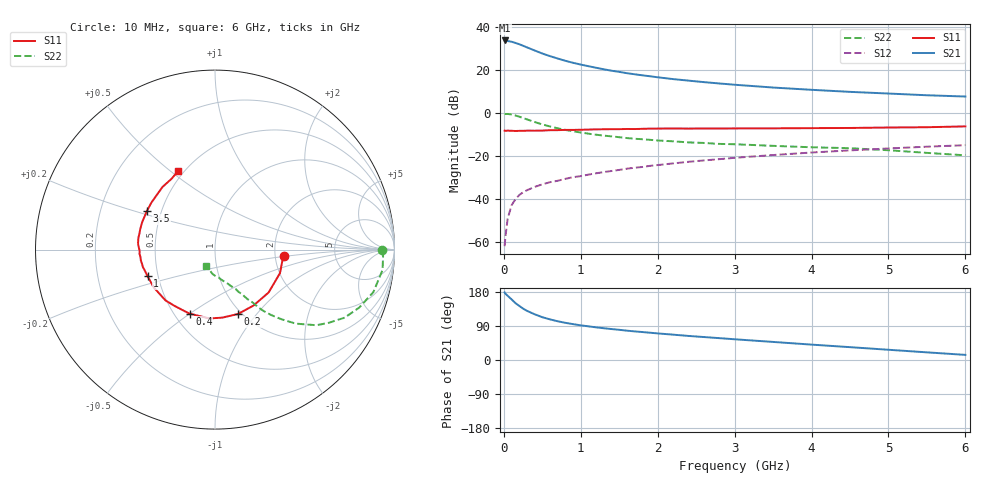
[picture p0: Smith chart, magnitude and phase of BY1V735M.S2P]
! SIEMENS Small Signal Semiconductors
! BFY420
! Si NPN RF SIEGET Grounded Emitter Transistor in MICRO-X
! VCE = 1.75 V  IC = 35 mA
! Common Emitter S-Parameters:  October  1996
# GHz  S  MA  R  50
!  f  S11  S21  S12  S22
! GHz  MAG  ANG  MAG  ANG  MAG  ANG  MAG  ANG
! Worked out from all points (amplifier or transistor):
!   36 points, 10 MHz to 6 GHz, reference 50 ohm
!   highest |S21| = 33.6 dB at 10 MHz (marker M1)
!   |S21| within 3 dB of that: start of sweep to 286.3 MHz
!   unconditionally stable (mu >= 1): start of sweep to 16.89 MHz; 1.433 GHz to end of sweep
!   at 250 MHz: K = 0.40, MSG = 34.0 dB, |S12| = -36.9 dB
!   at 1.4 GHz: K = 0.99, MSG = 23.3 dB, |S12| = -27.0 dB
!   at 6 GHz: K = 1.07, MAG = 9.7 dB, |S12| = -15.0 dB
!   S11 on the Smith chart (normalised r, x): 10 MHz: 2.24, -0.18; 200 MHz: 0.96, -0.81; 400 MHz: 0.60, -0.50; 1 GHz: 0.44, -0.15; 3.5 GHz: 0.42, +0.22; 6 GHz: 0.47, +0.53
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0.01  0.3852 -5.0  47.88 178.4  0.0008 112.9  0.9287 -0.3
0.02  0.3806 -8.9  47.52 175.1  0.0013 81.4  0.9372 -1.9
0.05  0.3851 -19.9  46.38 169.4  0.0035 85.0  0.9404 -6.9
0.1  0.3825 -38.6  44.77 160.1  0.0071 76.3  0.9137 -15.0
0.15  0.3784 -55.4  42 150.2  0.0098 72.3  0.866 -21.9
0.2  0.381 -70.4  39.2 142.9  0.0123 69.0  0.8157 -27.7
0.25  0.3812 -83.9  36.04 135.6  0.0143 66.5  0.7544 -32.7
0.3  0.3848 -94.5  33.12 129.8  0.0159 64.8  0.705 -36.7
0.4  0.3841 -111.7  28.03 120.7  0.019 62.3  0.6105 -42.5
0.5  0.3861 -125.5  23.82 112.9  0.0218 62.0  0.5373 -46.3
0.6  0.3953 -134.2  20.71 107.2  0.0245 61.5  0.4812 -49.3
0.7  0.3956 -142.3  18.24 102.2  0.0264 61.3  0.4372 -51.6
0.8  0.4016 -148.6  16.12 98.1  0.0293 60.8  0.4003 -53.2
1  0.4039 -158.5  13.17 91.5  0.0339 62.0  0.3487 -55.3
1.1  0.4078 -163.0  12.09 88.8  0.0367 62.0  0.3283 -56.8
1.4  0.4176 -171.7  9.488 81.7  0.0446 62.7  0.2835 -59.5
1.6  0.4212 -176.8  8.324 77.4  0.0504 61.6  0.2594 -61.6
2.2  0.4318 171.2  6.068 66.9  0.0668 59.3  0.2179 -67.0
3.5  0.4359 150.7  3.862 47.7  0.1045 50.5  0.1709 -78.2
4.5  0.4447 136.9  3.065 33.9  0.1341 41.7  0.1507 -87.4
5.5  0.4626 121.7  2.555 20.2  0.1634 31.9  0.1173 -104.5
6  0.4838 115.1  2.388 13.5  0.1771 27.0  0.103 -117.9
